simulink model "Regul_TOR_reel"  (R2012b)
settings: Solver=ode5  SolverMode=SingleTasking  StartTime=0.0  StopTime=inf  FixedStep=0.005  RelTol=1e-3  AbsTol=1e-6
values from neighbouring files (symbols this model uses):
  eta = 'a definir'    [assvt_TOR_init_.m]
undefined symbols (not defined in the file or in its folder): BaseAddress, T0

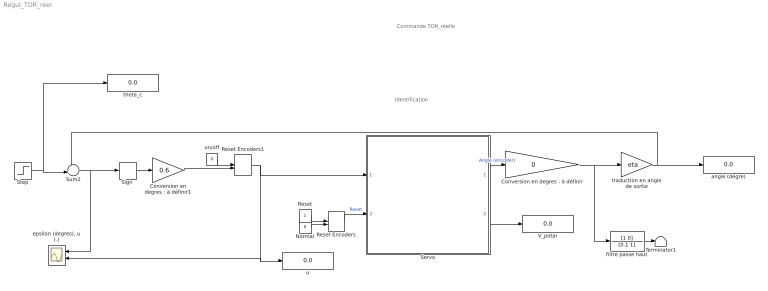
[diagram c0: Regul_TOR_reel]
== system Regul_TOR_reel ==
  note: Identification
  note: Commande TOR_réelle
  "Conversion en degres : à définir" : Gain  Gain=0
  "Conversion en degres : à définir1" : Gain  Gain=0.6
  Normal : Constant  Value=0
  Reset : Constant
  Reset Encoders : ManualSwitch  CurrentSetting=0
  Reset Encoders1 : ManualSwitch  CurrentSetting=0
  Servo : Subsystem
  Sign : Signum
  Step : Step  Time=10  After=45  SampleTime=0
  Sum2 : Sum  Inputs=-+|
  Terminator1 : Terminator
  V_potar : Display
  angle (degre) : Display
  "epsilon (degres), u (.)" : Scope  NumInputPorts=2
  filtre passe haut : TransferFcn  Numerator=[1 0]  Denominator=[0.1 1]
  on/off : Constant  Value=0
  theta_c : Display
  traduction en angle de sortie : Gain  Gain=eta
  u : Display
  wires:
  Reset Encoders/1 -> Servo/2(Reset Encoder)  "Reset"
  Normal/1 -> Reset Encoders/2
  Reset/1 -> Reset Encoders/1
  Servo/1(Codeur_angulaire) -> "Conversion en degres : à définir"/1  "Angle (encoder)"
  Sign/1 -> "Conversion en degres : à définir1"/1
  Servo/2(Set-up) -> V_potar/1
  Step/1 -> theta_c/1, Sum2/2
  Sum2/1 -> "epsilon (degres), u (.)"/1, Sign/1
  filtre passe haut/1 -> Terminator1/1
  "Conversion en degres : à définir"/1 -> filtre passe haut/1, traduction en angle de sortie/1
  traduction en angle de sortie/1 -> angle (degre)/1, Sum2/1
  on/off/1 -> Reset Encoders1/1
  Reset Encoders1/1 -> "epsilon (degres), u (.)"/2, u/1, Servo/1(PWM Control)
  "Conversion en degres : à définir1"/1 -> Reset Encoders1/2

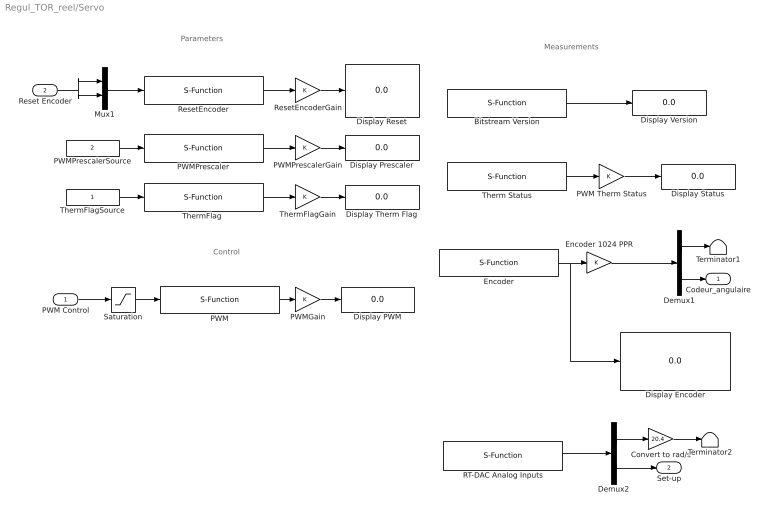
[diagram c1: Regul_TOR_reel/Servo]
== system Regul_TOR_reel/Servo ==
  note: Parameters
  note: Control
  note: Measurements
  PWM Control : Inport
  Reset Encoder : Inport  Port=2
  Bitstream Version : S-Function  FunctionName=Servo_BitstreamVersion  Parameters=BaseAddress, T0  EnableBusSupport=off
  Convert to rad/s : Gain  Gain=20.4
  Demux1 : Demux  Outputs=2
  Demux2 : Demux  Outputs=2
  Display Encoder : Display
  Display PWM : Display
  Display Prescaler : Display
  Display Reset : Display
  Display Status : Display
  Display Therm Flag : Display
  Display Version : Display
  Encoder : S-Function  FunctionName=Servo_Encoder  Parameters=BaseAddress, T0  EnableBusSupport=off
  Encoder 1024 PPR : Gain
  Mux1 : Mux  Inputs=2
  PWM : S-Function  FunctionName=Servo_PWM  Parameters=BaseAddress, T0  EnableBusSupport=off
  PWM Therm Status : Gain
  PWMGain : Gain
  PWMPrescaler : S-Function  FunctionName=Servo_PWMPrescaler  Parameters=BaseAddress, T0  EnableBusSupport=off
  PWMPrescalerGain : Gain
  PWMPrescalerSource : Constant  Value=2
  RT-DAC Analog Inputs : S-Function  FunctionName=servo_analoginputs  Parameters=BaseAddress, [1 0], [1 1], T0  EnableBusSupport=off
  ResetEncoder : S-Function  FunctionName=Servo_ResetEncoder  Parameters=BaseAddress, T0  EnableBusSupport=off
  ResetEncoderGain : Gain
  Saturation : Saturate  UpperLimit=1  LowerLimit=-1
  Terminator1 : Terminator
  Terminator2 : Terminator
  Therm Status : S-Function  FunctionName=Servo_PWMTherm  Parameters=BaseAddress, T0  EnableBusSupport=off
  "ThermFlag " : S-Function  FunctionName=Servo_ThermFlag  Parameters=BaseAddress, T0  EnableBusSupport=off
  ThermFlagGain : Gain
  ThermFlagSource : Constant
  Codeur_angulaire : Outport
  Set-up : Outport  Port=2
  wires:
  Encoder/1 -> Encoder 1024 PPR/1, Display Encoder/1
  Saturation/1 -> PWM/1
  PWM/1 -> PWMGain/1
  PWMGain/1 -> Display PWM/1
  ResetEncoder/1 -> ResetEncoderGain/1
  PWMPrescaler/1 -> PWMPrescalerGain/1
  Mux1/1 -> ResetEncoder/1
  PWMPrescalerSource/1 -> PWMPrescaler/1
  ResetEncoderGain/1 -> Display Reset/1
  PWMPrescalerGain/1 -> Display Prescaler/1
  PWM Control/1 -> Saturation/1
  Encoder 1024 PPR/1 -> Demux1/1
  Therm Status/1 -> PWM Therm Status/1
  PWM Therm Status/1 -> Display Status/1
  Bitstream Version/1 -> Display Version/1
  Reset Encoder/1 -> Mux1/1, Mux1/2
  "ThermFlag "/1 -> ThermFlagGain/1
  ThermFlagSource/1 -> "ThermFlag "/1
  ThermFlagGain/1 -> Display Therm Flag/1
  Demux1/1 -> Terminator1/1
  Demux1/2 -> Codeur_angulaire/1
  RT-DAC Analog Inputs/1 -> Demux2/1
  Demux2/2 -> Set-up/1
  Demux2/1 -> Convert to rad/s/1
  Convert to rad/s/1 -> Terminator2/1
